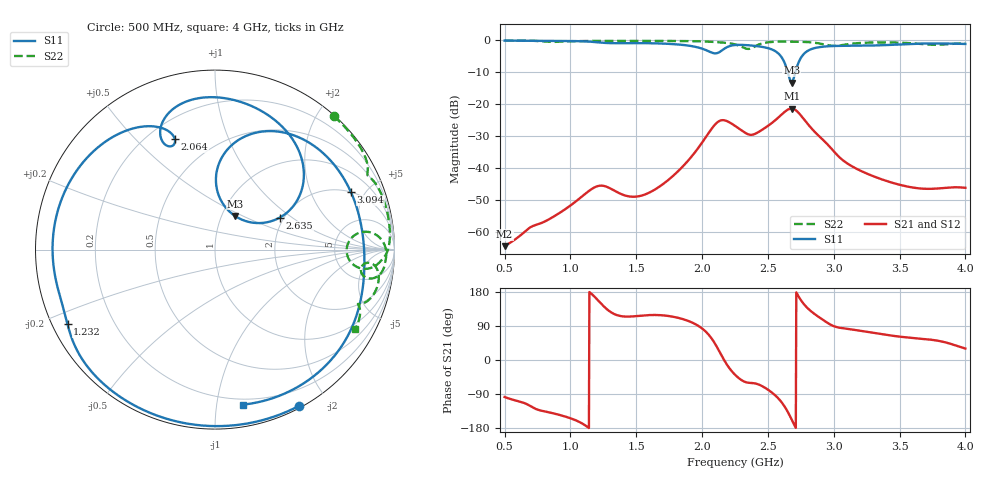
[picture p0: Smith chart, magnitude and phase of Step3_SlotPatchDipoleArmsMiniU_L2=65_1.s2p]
! TOUCHSTONE file generated by CST MICROWAVE STUDIO
! Date and time: Tue May 19 02:08:56 2020
! Project name: DualBand_DualMode_Antenna_FD_SteppedDesign.cst
! Parameters = {FPL=20; FPW=20; L=50; ST=10; SW=30; W=52; WF=7; ext=10; gap=1; inset=13}
! Header version: 2015
! Port assignment regex: !\s*Touchstone port\s*([0-9]+)\s*=\s*CST MWS port\s*([0-9]+)\s*\(\"(.*)\"\)(\s*mode\s*([0-9]+))?.*
! Touchstone port assignment:
! Touchstone port 1 = CST MWS port 1 ("")
! Touchstone port 2 = CST MWS port 2 ("")
# GHz S MA R 50
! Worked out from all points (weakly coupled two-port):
!   1006 points, 500 MHz to 4 GHz, reference 50 ohm
!   highest |S21| = -21.34 dB at 2.68 GHz (marker M1); lowest = -64.4 dB at 500 MHz (marker M2)
!   lowest |S11| = -13.2 dB at 2.68 GHz (marker M3), VSWR 1.56, Z = 57.9 + j22.7 ohm
!   |S11| at or under -10 dB: 2.651 GHz to 2.708 GHz (57.04 MHz wide, 2.13 % of centre)
!   |S22| runs from -2.7 to 0.0 dB; largest |S21 - S12| = 0.00019
!   S11 on the Smith chart (normalised r, x): 500 MHz: 0.02, -1.67; 1.232 GHz: 0.04, -0.24; 2.064 GHz: 0.31, +0.66; 2.635 GHz: 1.90, +0.81; 3.094 GHz: 1.99, +3.95; 4 GHz: 0.16, -1.18
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0.5  0.9886 -61.8  0.0006033 -97.7  0.0006034 -97.7  0.9956 48.3
0.794  0.9819 -98.0  0.00143 -134.9  0.001427 -135.2  0.9622 27.8
1.0845  0.9679 -134.7  0.003566 -166.6  0.003565 -166.2  0.9742 20.1
1.2315  0.9212 -153.1  0.005338 149.4  0.005353 149.5  0.98 16.0
1.4695  0.905 -179.0  0.003578 115.0  0.003554 115.3  0.9819 10.6
1.669  0.8947 156.3  0.005036 118.5  0.005032 118.7  0.98 6.6
1.9  0.825 126.3  0.01359 102.4  0.01359 102.3  0.9718 2.0
2.0645  0.6541 110.0  0.03926 60.5  0.03925 60.5  0.95 -1.9
2.1695  0.741 114.2  0.05614 -1.4  0.05614 -1.4  0.9182 -4.5
2.25  0.844 99.4  0.04595 -38.9  0.04594 -38.9  0.8652 -7.0
2.376  0.8294 77.4  0.03326 -60.7  0.03327 -60.7  0.7547 4.2
2.523  0.7295 50.9  0.04965 -84.0  0.04965 -84.0  0.9415 2.1
2.586  0.6046 36.0  0.06383 -104.0  0.06383 -104.0  0.9539 -0.6
2.635  0.4025 26.3  0.07828 -127.3  0.07829 -127.3  0.9545 -2.4
2.6805  0.2181 59.0  0.08568 -157.1  0.08574 -157.1  0.9521 -3.8
2.7365  0.4689 87.8  0.07219 165.6  0.07235 165.6  0.9488 -5.4
2.8345  0.7352 63.8  0.04121 126.7  0.04133 126.5  0.9266 -8.7
2.95  0.8057 42.7  0.02391 98.6  0.02385 98.3  0.8439 -10.2
3.0935  0.8222 23.1  0.01224 82.7  0.01225 82.6  0.8619 -4.9
3.419  0.8471 -12.7  0.006148 65.3  0.00616 65.3  0.9269 -13.1
3.6675  0.8903 -40.9  0.004798 56.0  0.0048 56.0  0.8762 -20.0
4  0.8777 -79.8  0.004936 30.2  0.004937 30.2  0.8982 -29.4
